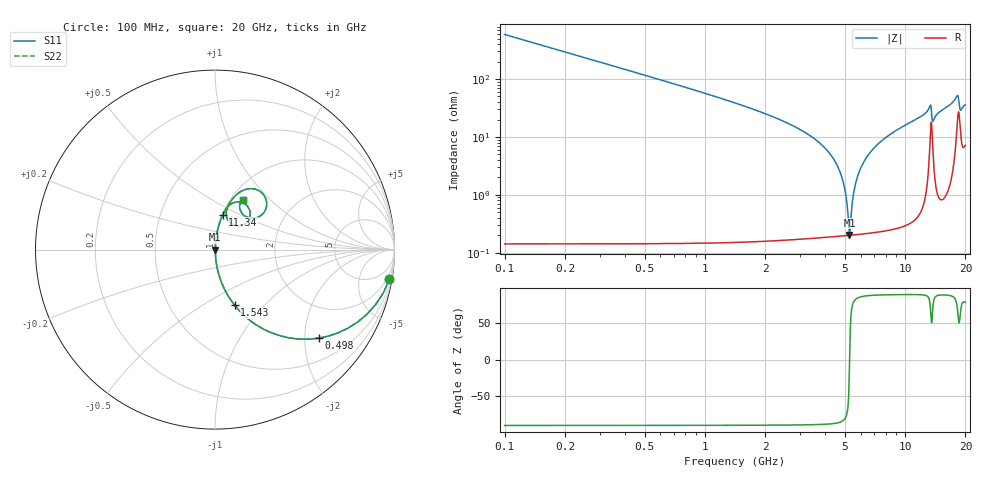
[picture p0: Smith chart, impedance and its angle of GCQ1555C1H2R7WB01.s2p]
!Murata Part Number: GCQ1555C1H2R7WB01
!These Parameters are Measured in Series Mode Connection
!Data Generated on Jan 08, 2026
!  o--ll--o
!Port1  Port2
!  o------o
!Operation Temp=25[degC], DC Bias Voltage=0[V]
!Freq. Start=100[MHz] Stop=20[GHz] 401[Steps]
# Hz S RI R 50
!Freq.(Hz) S11(Real) S11(Imag) S21(Real) S21(Imag) S12(Real) S12(Imag) S22(Real) S22(Imag)
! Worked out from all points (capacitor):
!   401 points, 100 MHz to 20 GHz, reference 50 ohm
!   read as one part in series: C = 2.7 pF near 199.5 MHz
!   lowest |Z| = 203 mohm at 5.274 GHz (marker M1)
!   series resonance near 5.282 GHz, so ESL is about 340 pH
!   S11 on the Smith chart (normalised r, x): 100 MHz: 1, -12; 498 MHz: 1.00, -2.35; 1.543 GHz: 1.00, -0.70; 11.34 GHz: 1.01, +0.40; 20 GHz: 1.14, +0.70
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1e8  0.972 -0.1649  0.028 0.1649  0.028 0.1649  0.972 -0.1649
2.99e8  0.7941 -0.404  0.2059 0.404  0.2059 0.404  0.7941 -0.404
4.98e8  0.5791 -0.4931  0.4209 0.4931  0.4209 0.4931  0.5791 -0.4931
9.4575e8  0.2674 -0.4414  0.7326 0.4414  0.7326 0.4414  0.2674 -0.4414
1.54275e9  0.11 -0.3107  0.89 0.3107  0.89 0.3107  0.11 -0.3107
3.43325e9  0.0115 -0.0981  0.9885 0.0981  0.9885 0.0981  0.0115 -0.0981
4.22925e9  0.00437 -0.0499  0.9956 0.0499  0.9956 0.0499  0.00437 -0.0499
4.72675e9  0.00255 -0.0249  0.9975 0.0249  0.9975 0.0249  0.00255 -0.0249
4.9755e9  0.00214 -0.0134  0.9979 0.0134  0.9979 0.0134  0.00214 -0.0134
5.274e9  0.002 -0.000329  0.998 0.000329  0.998 0.000329  0.002 -0.000329
5.3735e9  0.00202 0.00386  0.998 -0.00386  0.998 -0.00386  0.00202 0.00386
5.5725e9  0.00218 0.012  0.9978 -0.012  0.9978 -0.012  0.00218 0.012
5.7715e9  0.00245 0.0199  0.9975 -0.0199  0.9975 -0.0199  0.00245 0.0199
6.7665e9  0.00536 0.0562  0.9946 -0.0562  0.9946 -0.0562  0.00536 0.0562
1.005e10  0.0279 0.1559  0.9721 -0.1559  0.9721 -0.1559  0.0279 0.1559
1.13435e10  0.0427 0.1928  0.9573 -0.1928  0.9573 -0.1928  0.0427 0.1928
1.338325e10  0.1797 0.2438  0.8203 -0.2438  0.8203 -0.2438  0.1797 0.2438
1.37315e10  0.0877 0.1466  0.9123 -0.1466  0.9123 -0.1466  0.0877 0.1466
1.67165e10  0.1235 0.3091  0.8765 -0.3091  0.8765 -0.3091  0.1235 0.3091
1.835825e10  0.2882 0.26  0.7118 -0.26  0.7118 -0.26  0.2882 0.26
1.885575e10  0.1647 0.1888  0.8353 -0.1888  0.8353 -0.1888  0.1647 0.1888
2e10  0.1567 0.2754  0.8433 -0.2754  0.8433 -0.2754  0.1567 0.2754
